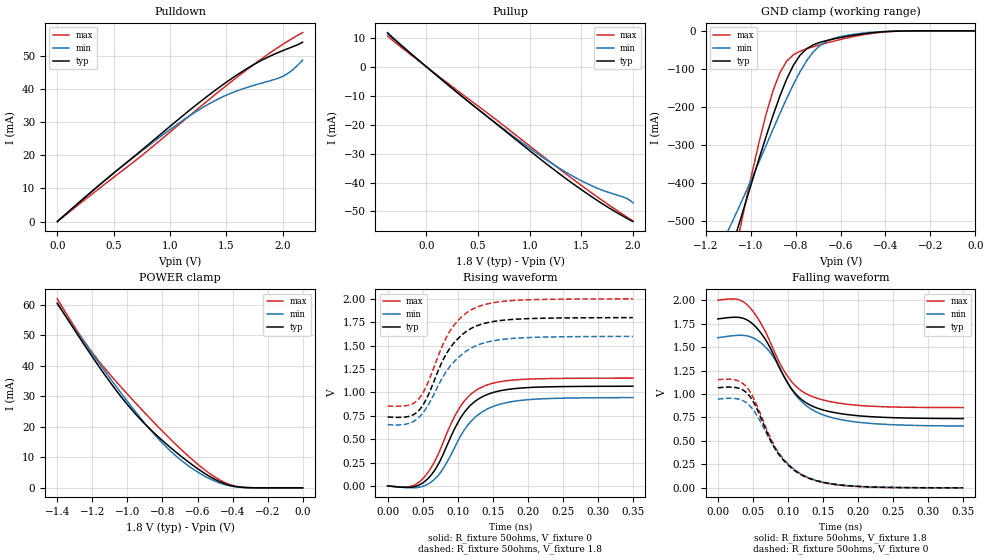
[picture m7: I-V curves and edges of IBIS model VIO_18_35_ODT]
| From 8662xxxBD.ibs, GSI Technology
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|  signals   DQA1-DQA9, DQB1-DQB9, DQC1-DQC9, DQD1-DQD9
[Model]   VIO_18_35_ODT
Model_type   I/O
Polarity   Non-Inverting
Vinl  =   0.7000V
Vinh  =   1.1000V
Vmeas =   0.90v
Rref  =   50
|  variable   typ   min   max
C_comp   3.0pF   2.5pF   3.5pF
[Receiver Thresholds]
Vth = 0.90V
Vth_min = 0.80V
Vth_max = 0.95V
Threshold_sensitivity = 1.0
Reference_supply Ext_ref
Vinh_ac = +200mv
Vinh_dc = +100mv
Vinl_ac = -200mv
Vinl_dc = -100mv
Tslew_ac = 550ps
|  variable   typ   min   max
[External Reference]   0.90   0.80   0.95
|  variable   typ   min   max
[Temperature Range]   50   100   0
|  variable   typ   min   max
[Voltage Range]   1.8   1.6   2.0
[Add Submodel]
| Submodel Name   Mode
Strong_ODT_15V   Non-Driving
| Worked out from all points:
|   slope of the pulldown table from 0 to 0.27 V, typ, clamps not added: 33.7 ohm
|   slope of the pullup table from 0 to 0.27 V, typ, clamps not added: 33.6 ohm
|   GND clamp passes 1 mA (typ) near -0.36 V on its own axis
|   POWER clamp passes 1 mA (typ) near -0.43 V on its own axis
|   rising waveform, R_fixture 50ohms, V_fixture 0: 20-80 % time 46.1ps typ, 48.7ps min, 46.2ps max; typ from 0 V to 1.06 V
|   rising waveform, R_fixture 50ohms, V_fixture 1.8: 20-80 % time 45.4ps typ, 50.5ps min, 44.4ps max; typ from 0.737 V to 1.8 V
|   falling waveform, R_fixture 50ohms, V_fixture 1.8: 20-80 % time 50.7ps typ, 54ps min, 51.2ps max; typ from 1.8 V to 0.738 V
|   falling waveform, R_fixture 50ohms, V_fixture 0: 20-80 % time 49.6ps typ, 53.2ps min, 50.5ps max; typ from 1.07 V to 0 V
[Pullup]
| V(VDDQ-Vout)   typ   min   max
-376mV    11.62mA    11.84mA    10.71mA
-280mV    8.498mA    8.685mA    7.759mA
-16mV     482uA      488.8uA    441.6uA
368mV     -10.89mA   -10.92mA   -10.03mA
776mV     -22.56mA   -22.22mA   -21.07mA
1.088V    -31.46mA   -30.35mA   -29.81mA
1.304V    -37.38mA   -35.41mA   -35.75mA
1.496V    -42.35mA   -39.3mA    -40.87mA
1.688V    -46.96mA   -42.43mA   -45.8mA
1.928V    -52.1mA    -45.32mA   -51.62mA
2V        -53.5mA    -46.99mA   -53.28mA
[PullDown]
| voltage   typ   min   max
0V        -7.795nA   -15.24nA   -7.985nA
286mV     8.485mA    8.587mA    7.716mA
550mV     16.03mA    16.03mA    14.67mA
946mV     27.21mA    26.43mA    25.49mA
1.188V    34.01mA    32.25mA    32.39mA
1.32V     37.55mA    35.03mA    36.11mA
1.452V    40.92mA    37.43mA    39.76mA
1.694V    46.43mA    40.63mA    46.18mA
1.848V    49.31mA    42.15mA    50.01mA
2.002V    51.65mA    43.89mA    53.55mA
2.09V     52.83mA    45.87mA    55.4mA
2.178V    54.19mA    48.77mA    57.1mA
[POWER Clamp]
|V(VDDQ-Vout)   typ   min   max
-1.4V     60.61mA    60.34mA    62.02mA
-1.288V   50.59mA    51.1mA     51.64mA
-1.204V   43.31mA    44.28mA    44.66mA
-1.008V   27.88mA    28.96mA    31.27mA
-924mV    22.38mA    22.81mA    26.03mA
-812mV    16.12mA    15.39mA    19.29mA
-672mV    9.383mA    8.076mA    11.45mA
-588mV    5.846mA    4.807mA    7.253mA
-504mV    2.89mA     2.285mA    3.677mA
-392mV    517.1uA    405.4uA    668.9uA
-308mV    61.99uA    56.59uA    69.17uA
0V        31.94nA    55.59nA    13.84nA
[GND Clamp]
|(Vout)   typ   min   max
-1.5V     -1.252A    -991.4mA   -1.695A
-1.11V    -618mA     -537.1mA   -698.9mA
-1.08V    -561.6mA   -499.5mA   -613.1mA
-1.05V    -504.3mA   -461mA     -527.9mA
-930mV    -275.4mA   -299.5mA   -216.8mA
-900mV    -221.7mA   -258.3mA   -156.7mA
-870mV    -171.8mA   -217.7mA   -110.4mA
-810mV    -90.76mA   -141.2mA   -63.07mA
-720mV    -36.41mA   -54.52mA   -41.49mA
-630mV    -21.21mA   -19.75mA   -26.99mA
-390mV    -1.828mA   -1.276mA   -2.431mA
0V        -7.821nA   -15.24nA   -8.228nA
[Ramp]
| voltage   typ   min   max
dV/dt_r   0.54/186p   0.48/213p   0.60/209p
dV/dt_f   0.86/129p   0.66/166p   1.07/101p
R_load  =   50ohms
[Rising Waveform]
R_fixture =   50ohms
V_fixture =   0
| Time   V(typ)   V(min)   V(max)
0s        155.5nV    299.8nV    169nV
35ps      -12.37mV   -20.8mV    -849.5uV
56ps      67.19mV    13.28mV    128mV
77ps      301.5mV    159.7mV    424.2mV
91ps      537.9mV    342.2mV    672.8mV
105ps     737.8mV    545.5mV    862mV
119ps     867.3mV    690.8mV    981.5mV
136.5ps   957.8mV    798.1mV    1.063V
196ps     1.049V     918.4mV    1.14V
350ps     1.065V     944.1mV    1.152V
[Rising Waveform]
R_fixture =   50ohms
V_fixture =   1.8
V_fixture_min =  1.6
V_fixture_max =  2.0
| Time   V(typ)   V(min)   V(max)
0s        737.4mV    656.3mV    854.9mV
31.5ps    745.3mV    670.7mV    865.6mV
45.5ps    813.8mV    738.2mV    939.7mV
56ps      940.1mV    841mV      1.078V
77ps      1.314V     1.14V      1.478V
87.5ps    1.457V     1.263V     1.638V
105ps     1.608V     1.399V     1.804V
126ps     1.707V     1.498V     1.906V
189ps     1.784V     1.581V     1.986V
350ps     1.799V     1.598V     1.999V
[Falling Waveform]
R_fixture =   50ohms
V_fixture =   1.8
V_fixture_min = 1.6
V_fixture_max = 2.0
| Time   V(typ)   V(min)   V(max)
0s        1.8V       1.6V       2V
35ps      1.809V     1.625V     1.988V
59.5ps    1.668V     1.556V     1.776V
80.5ps    1.401V     1.38V      1.453V
101.5ps   1.095V     1.094V     1.167V
115.5ps   967.1mV    949.5mV    1.055V
133ps     877.1mV    839.8mV    977.8mV
161ps     810mV      751.9mV    918.1mV
199.5ps   769mV      700mV      879.6mV
350ps     738.4mV    658.6mV    855.3mV
[Falling Waveform]
R_fixture =   50ohms
V_fixture =   0
| Time   V(typ)   V(min)   V(max)
0s        1.067V     945.8mV    1.153V
24.5ps    1.07V      952.1mV    1.15V
38.5ps    1.029V     918.1mV    1.094V
52.5ps    891.7mV    810mV      931.9mV
73.5ps    533.6mV    519.8mV    557.8mV
87.5ps    350.7mV    355.9mV    366.7mV
105ps     210.9mV    219.8mV    220.6mV
126ps     113.3mV    120mV      117.7mV
189ps     20.27mV    23.37mV    18.65mV
350ps     305.2uV    564.9uV    164.8uV
